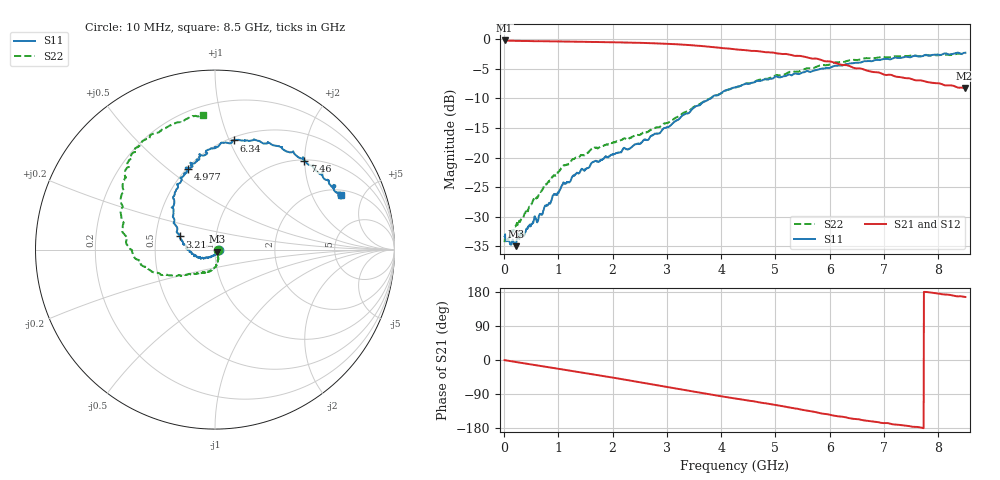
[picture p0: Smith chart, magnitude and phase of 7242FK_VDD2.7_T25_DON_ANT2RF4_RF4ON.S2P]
!Agilent Technologies,E5071C,MY46417908,A.11.23
!Date: Wed Dec 09 15:40:08 2020
!Data & Calibration Information:
!Freq	S11:SOLT2(ON)	S21:SOLT2(ON)	S12:SOLT2(ON)	S22:SOLT2(ON)
!PortZ  Port1:50+j0  Port2:50+j0
!Above PortZ is port z conversion or system Z0 setting when saving the data.
!When reading, reference impedance value at option line is always used.
# Hz S dB R 50
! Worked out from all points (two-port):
!   1601 points, 10 MHz to 8.5 GHz, reference 50 ohm
!   highest |S21| = -0.23 dB at 10 MHz (marker M1); lowest = -8.3 dB at 8.484 GHz (marker M2)
!   |S21| within 3 dB of the highest: start of sweep to 5.649 GHz
!   lowest |S11| = -34.9 dB at 216.9 MHz (marker M3), VSWR 1.04, Z = 51.4 - j1.19 ohm
!   |S11| at or under -10 dB: start of sweep to 3.812 GHz
!   |S22| runs from -34.3 to -2.4 dB; largest |S21 - S12| = 0.0055
!   S11 on the Smith chart (normalised r, x): 10 MHz: 1.04, -0.00; 3.21 GHz: 0.67, +0.10; 4.977 GHz: 0.51, +0.59; 6.34 GHz: 0.53, +1.04; 7.46 GHz: 1.02, +1.99; 8.5 GHz: 2.30, +3.38
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1e7  -33.31 -0.3  -0.23 -0.4  -0.23 -0.4  -34.27 -8.5
1.002062e8  -34.19 -22.3  -0.28 -2.5  -0.27 -2.5  -33.41 -24.4
2.169438e8  -34.95 -40.1  -0.30 -5.3  -0.30 -5.2  -31.50 -39.9
6.414438e8  -29.83 -99.1  -0.35 -15.0  -0.35 -15.0  -26.15 -68.2
7.741e8  -28.16 -110.6  -0.37 -18.0  -0.37 -18.0  -24.55 -74.4
1.081862e9  -24.48 -131.5  -0.41 -25.0  -0.41 -25.0  -21.50 -84.0
1.426769e9  -21.94 -142.6  -0.46 -33.1  -0.46 -33.1  -19.56 -94.8
1.654938e9  -20.67 -147.7  -0.49 -38.3  -0.49 -38.3  -18.40 -101.6
2.1325e9  -19.12 -160.5  -0.56 -49.6  -0.56 -49.6  -17.15 -113.7
2.843538e9  -15.95 176.1  -0.72 -66.9  -0.73 -66.9  -14.87 -132.0
3.209669e9  -13.59 159.5  -0.89 -76.1  -0.89 -76.1  -13.06 -140.1
3.857031e9  -9.62 135.5  -1.36 -92.2  -1.35 -92.2  -9.65 -154.6
4.255e9  -8.15 124.2  -1.73 -101.5  -1.72 -101.5  -8.17 -164.6
4.97665e9  -6.48 108.6  -2.31 -118.3  -2.30 -118.4  -6.26 177.5
5.671769e9  -5.44 94.9  -3.29 -135.8  -3.24 -135.8  -4.92 154.9
6.340356e9  -4.19 80.3  -4.45 -153.0  -4.47 -152.7  -3.62 139.7
6.664038e9  -3.73 69.7  -5.25 -159.9  -5.27 -159.8  -3.24 134.3
7.088538e9  -3.38 56.6  -6.00 -167.1  -6.06 -167.2  -3.06 129.4
7.459975e9  -3.06 44.9  -6.62 -174.1  -6.61 -174.1  -2.83 124.7
7.942844e9  -2.63 31.6  -7.41 176.6  -7.44 176.8  -2.72 114.0
8.484081e9  -2.32 22.8  -8.27 166.6  -8.39 166.5  -2.49 95.9
8.5e9  -2.30 23.3  -8.25 166.3  -8.35 166.3  -2.45 95.3
